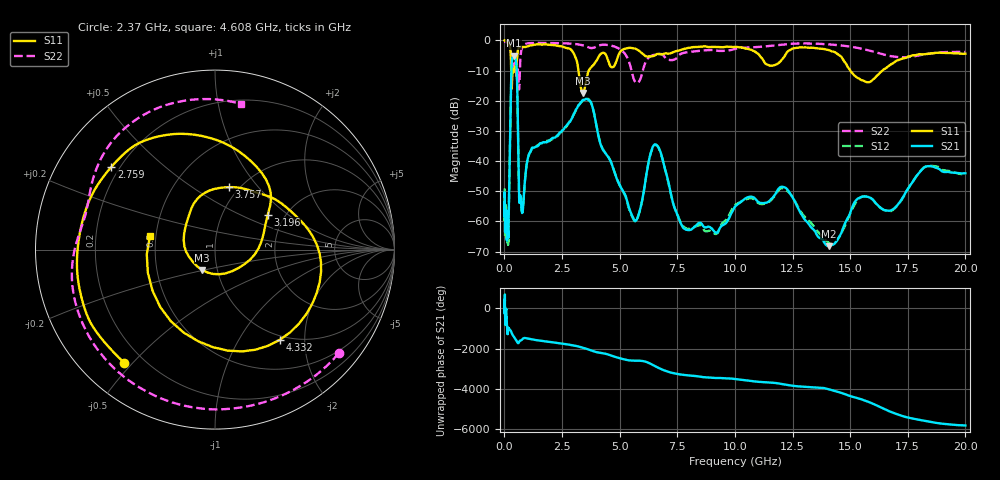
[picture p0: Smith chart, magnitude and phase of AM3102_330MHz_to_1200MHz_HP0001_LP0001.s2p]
! Date/Time: Tue, Sep 11, 2018 5:09 PM
! Network Analyzer: Agilent Technologies E8362B Rev: A.07.50.63
! Sweep from 0.010 to 20.000 GHz, 1601 Points, Sweep Type: LOG
! Power Supply: 4.950 V, 0.001 A
# Hz S DB R 50
!freq MagS11 AngS11 MagS21 AngS21 MagS12 AngS12 MagS22 AngS22
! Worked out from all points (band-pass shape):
!   1601 points, 10 MHz to 20 GHz, reference 50 ohm
!   highest |S21| = -5.03 dB at 402.8 MHz (marker M1); lowest = -68.2 dB at 14.07 GHz (marker M2)
!   |S21| within 3 dB of the highest: 316.3 MHz to 520.9 MHz (204.6 MHz wide, 48.9 % of centre)
!   lowest |S11| = -17.4 dB at 3.416 GHz (marker M3), VSWR 1.31, Z = 42.3 - j9.75 ohm
!   |S11| at or under -10 dB: 295.7 MHz to 354.9 MHz (59.21 MHz wide, 18.2 % of centre); 3.211 GHz to 3.66 GHz (448.9 MHz wide, 13.1 % of centre); 15.01 GHz to 16.4 GHz (1.393 GHz wide, 8.87 % of centre)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
!   |S22| runs from -16.3 to -0.2 dB; largest |S21 - S12| = 0.0076
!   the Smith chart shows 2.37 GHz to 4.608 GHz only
!   S11 on the Smith chart (normalised r, x): 2.37 GHz: 0.13, -0.47; 2.759 GHz: 0.17, +0.34; 3.196 GHz: 1.63, +0.72; 3.757 GHz: 0.90, +0.71; 4.332 GHz: 0.93, -1.52; 4.608 GHz: 0.46, +0.08
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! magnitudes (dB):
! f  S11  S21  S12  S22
! 10 MHz  0.0  -51.6  -52.2  -0.3
! 35.55 MHz  0.0  -61.2  -61.1  -0.4
! 126.4 MHz  -0.4  -63.4  -64.3  -0.8
! 174.6 MHz  -0.9  -63.5  -63.0  -1.1
! 305.8 MHz  -14.0  -10.0  -10.0  -6.7
! 402.8 MHz  -10.5  -5.0  -5.1  -8.3
! 447.2 MHz  -8.9  -5.5  -5.5  -7.4
! 761.4 MHz  -2.1  -57.1  -56.7  -2.5
! 1.59 GHz  -1.4  -34.0  -34.0  -0.8
! 2.37 GHz  -1.9  -30.8  -31.2  -0.9
! 2.759 GHz  -2.6  -27.7  -27.8  -1.0
! 3.196 GHz  -9.1  -21.6  -21.9  -1.3
! 3.416 GHz  -17.4  -19.7  -19.9  -1.6
! 3.757 GHz  -9.0  -20.6  -20.6  -2.5
! 4.332 GHz  -4.2  -36.8  -36.8  -1.4
! 4.608 GHz  -8.6  -40.0  -40.0  -1.7
! 5.652 GHz  -2.7  -59.7  -59.9  -13.5
! 6.58 GHz  -4.7  -34.5  -34.7  -4.6
! 7.882 GHz  -2.6  -62.8  -62.3  -4.0
! 12.09 GHz  -5.9  -48.6  -49.0  -1.3
! 14.07 GHz  -3.2  -68.2  -67.1  -1.3
! 20 GHz  -4.4  -44.0  -44.6  -3.8
